(* Logix 5000 AddOnInstructionDefinition export P42_AOI_4P; software revision 33.00 *)

ADD_ON_INSTRUCTION P42_AOI_4P   (* revision 1.0, vendor PM Controls *)
// Anderson-Negele Pressure Transmitter
// Revision note:
// psm
// Help:
// Input_PressureUnit_INT controls the Process Data conversion. The value needs to be equal with the parameter value of "Pressure unit" (Index 212):
// 0: [bar]
// 1: [mbar]
// 2: [psi]
// 3:[MPa]
VAR_OUTPUT
   IOLink_Mode : BOOL; {access Read Only, visible}
END_VAR
VAR_IN_OUT
   Input : INT[123]; {required}
END_VAR
VAR_INPUT
   Input_PressureUnit_INT : INT; {visible}
   Port_Process_Data_Size : DINT;
   Port_Number : INT; {visible}
END_VAR
VAR_OUTPUT
   Device_Not_Connected : BOOL; {access Read Only, visible}
   Vendor_ID : INT; {access Read Only, visible}
   Device_ID : DINT; {access Read Only, visible}
   Invalid_Data : BOOL; {access Read Only, visible}
   Pressure : REAL; {access Read Only, visible}
END_VAR
VAR
   Data_Size : INT; {access None}
   RealPort_Num : INT; {access None}
   Offset_Address : INT; {access None}
   Process_Offset : INT; {access None}
   StatusFlgs_Offset : INT; {access None}
   Offset_StatusFlgs : INT; {access None}
   PD_Right_Shift_Value : INT := 4; {access None}
   PD_Value : INT; {access None}
   Pressure_Value_Gradient : REAL := 0.001; {access Read Only}
   GradientClass1 : BOOL; {access None}
   GradientClass2 : BOOL; {access None}
   GradientClass3 : BOOL; {access None}
   Pressure_Value_Gradient_Unit : REAL; {access None}
END_VAR

ROUTINE Logic   (* ladder *)
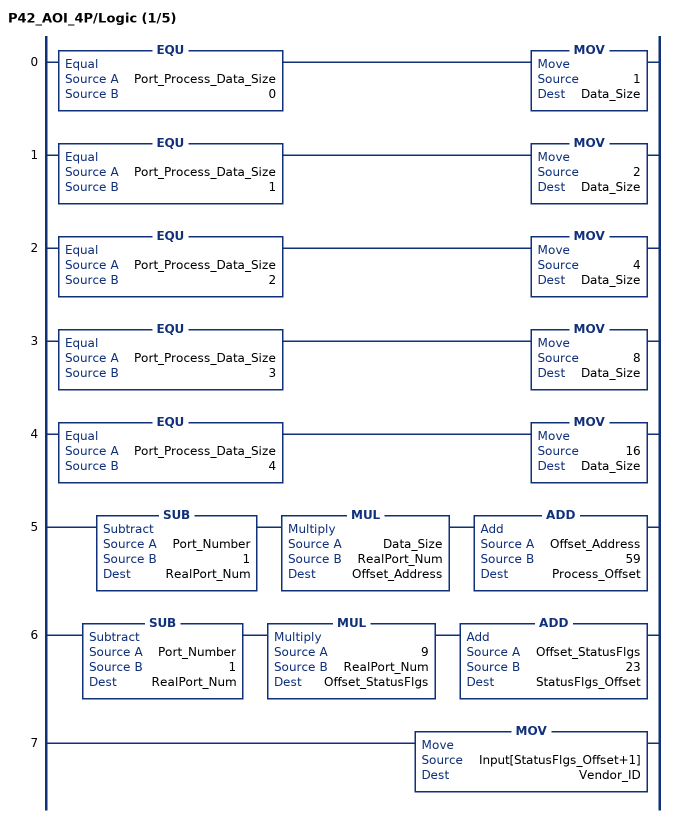
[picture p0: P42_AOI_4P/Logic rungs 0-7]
   0: EQU(Port_Process_Data_Size,0)MOV(1,Data_Size);
   1: EQU(Port_Process_Data_Size,1)MOV(2,Data_Size);
   2: EQU(Port_Process_Data_Size,2)MOV(4,Data_Size);
   3: EQU(Port_Process_Data_Size,3)MOV(8,Data_Size);
   4: EQU(Port_Process_Data_Size,4)MOV(16,Data_Size);
   5: SUB(Port_Number,1,RealPort_Num)MUL(Data_Size,RealPort_Num,Offset_Address)ADD(Offset_Address,59,Process_Offset);
   6: SUB(Port_Number,1,RealPort_Num)MUL(9,RealPort_Num,Offset_StatusFlgs)ADD(Offset_StatusFlgs,23,StatusFlgs_Offset);
   7: MOV(Input[StatusFlgs_Offset+1],Vendor_ID);
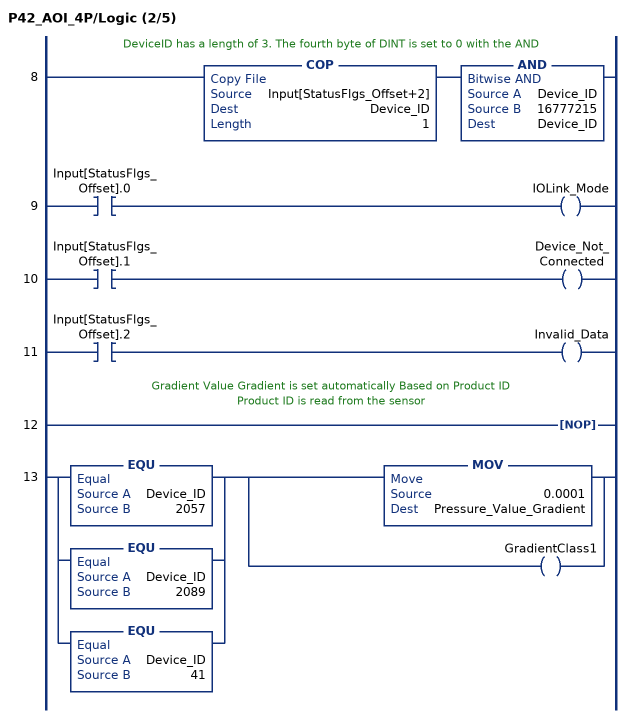
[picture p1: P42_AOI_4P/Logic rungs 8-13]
   // DeviceID has a length of 3. The fourth byte of DINT is set to 0 with the AND
   8: COP(Input[StatusFlgs_Offset+2],Device_ID,1)AND(Device_ID,16777215,Device_ID);
   9: XIC(Input[StatusFlgs_Offset].0)OTE(IOLink_Mode);
   10: XIC(Input[StatusFlgs_Offset].1)OTE(Device_Not_Connected);
   11: XIC(Input[StatusFlgs_Offset].2)OTE(Invalid_Data);
   // Gradient Value Gradient is set automatically Based on Product ID
   // Product ID is read from the sensor
   12: NOP();
   13: [EQU(Device_ID,2057) ,EQU(Device_ID,2089) ,EQU(Device_ID,41) ][MOV(0.0001,Pressure_Value_Gradient) ,OTE(GradientClass1) ];
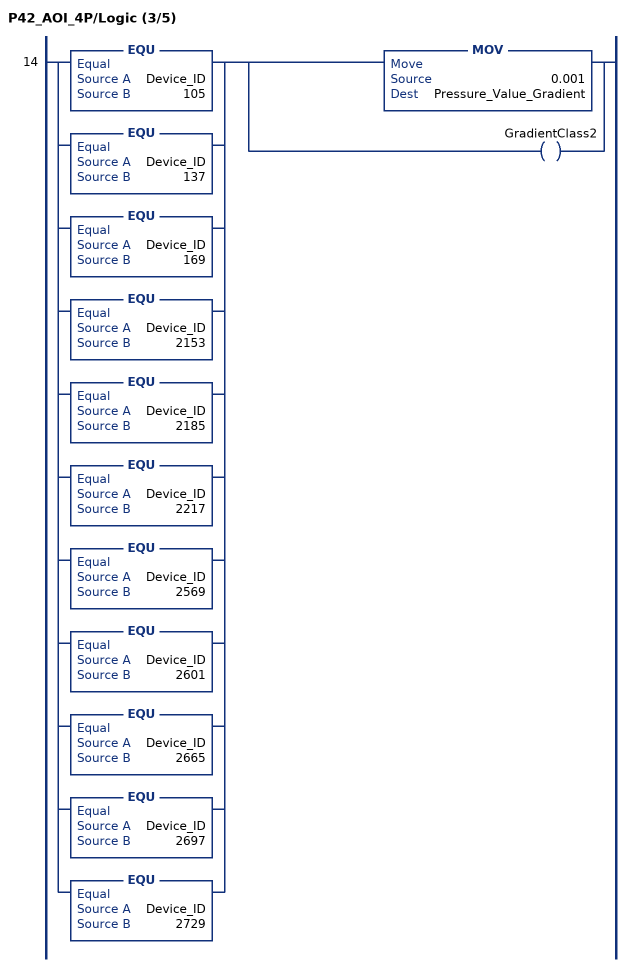
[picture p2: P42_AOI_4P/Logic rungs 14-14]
   14: [EQU(Device_ID,105) ,EQU(Device_ID,137) ,EQU(Device_ID,169) ,EQU(Device_ID,2153) ,EQU(Device_ID,2185) ,EQU(Device_ID,2217) ,EQU(Device_ID,2569) ,EQU(Device_ID,2601) ,EQU(Device_ID,2665) ,EQU(Device_ID,2697) ,EQU(Device_ID,2729) ][MOV(0.001,Pressure_Value_Gradient) ,OTE(GradientClass2) ];
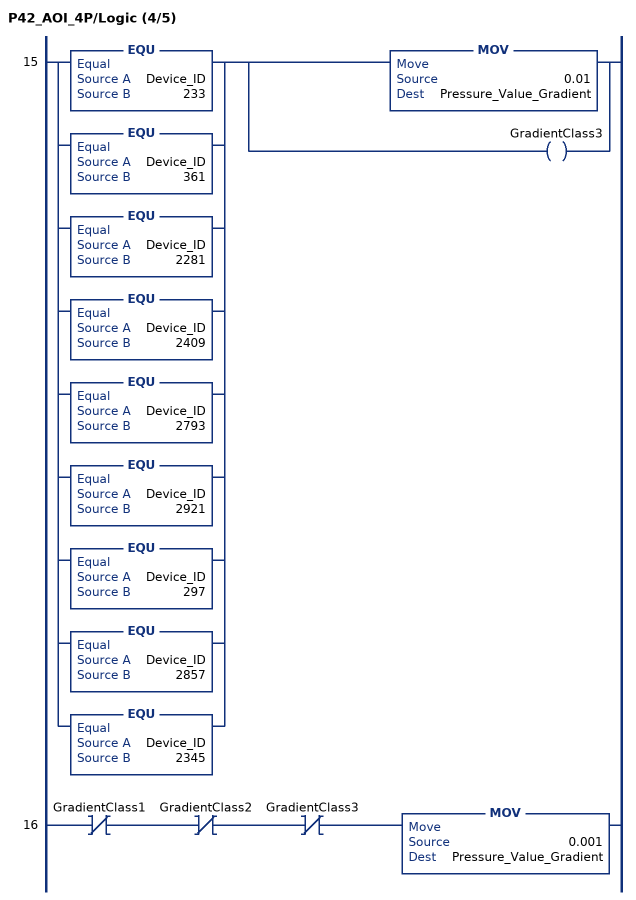
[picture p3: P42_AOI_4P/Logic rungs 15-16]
   15: [EQU(Device_ID,233) ,EQU(Device_ID,361) ,EQU(Device_ID,2281) ,EQU(Device_ID,2409) ,EQU(Device_ID,2793) ,EQU(Device_ID,2921) ,EQU(Device_ID,297) ,EQU(Device_ID,2857) ,EQU(Device_ID,2345) ][MOV(0.01,Pressure_Value_Gradient) ,OTE(GradientClass3) ];
   16: XIO(GradientClass1)XIO(GradientClass2)XIO(GradientClass3)MOV(0.001,Pressure_Value_Gradient);
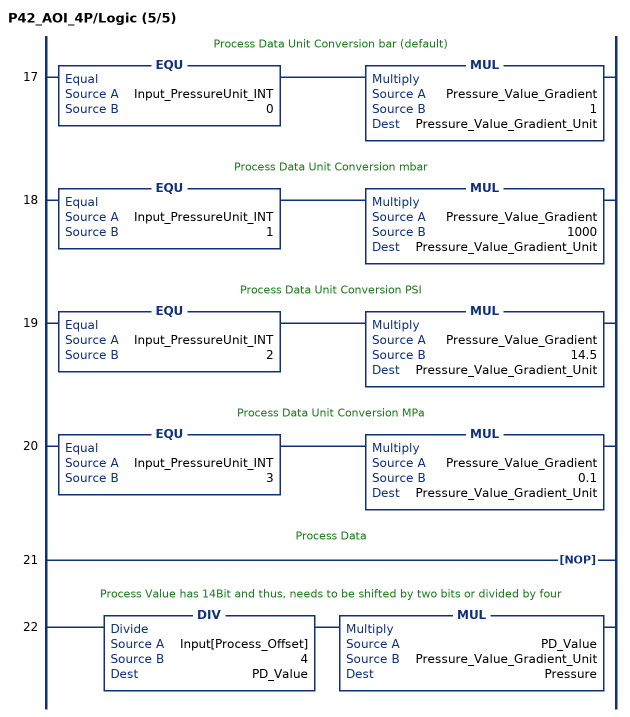
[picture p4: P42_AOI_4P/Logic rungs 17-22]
   // Process Data Unit Conversion bar (default)
   17: EQU(Input_PressureUnit_INT,0)MUL(Pressure_Value_Gradient,1,Pressure_Value_Gradient_Unit);
   // Process Data Unit Conversion mbar
   18: EQU(Input_PressureUnit_INT,1)MUL(Pressure_Value_Gradient,1000,Pressure_Value_Gradient_Unit);
   // Process Data Unit Conversion PSI
   19: EQU(Input_PressureUnit_INT,2)MUL(Pressure_Value_Gradient,14.5,Pressure_Value_Gradient_Unit);
   // Process Data Unit Conversion MPa
   20: EQU(Input_PressureUnit_INT,3)MUL(Pressure_Value_Gradient,0.1,Pressure_Value_Gradient_Unit);
   // Process Data
   21: NOP();
   // Process Value has 14Bit and thus, needs to be shifted by two bits or divided by four
   22: DIV(Input[Process_Offset],4,PD_Value)MUL(PD_Value,Pressure_Value_Gradient_Unit,Pressure);
END_ROUTINE
END_ADD_ON_INSTRUCTION
